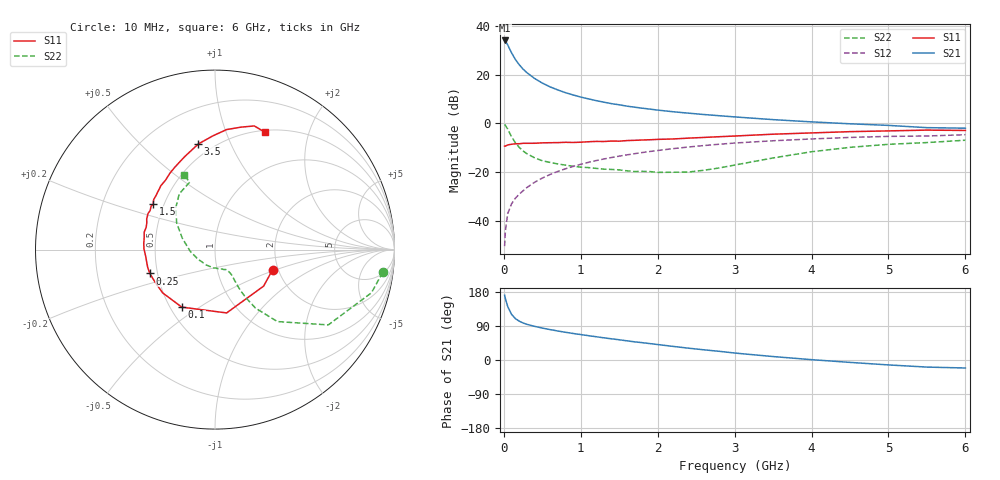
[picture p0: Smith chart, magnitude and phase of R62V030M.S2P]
! SIEMENS Small Signal Semiconductors
! BFR193
! Si NPN RF Bipolar Junction Transistor in SOT23
! VCE = 2 V  IC = 30 mA
! Common Emitter S-Parameters:  May  1996
# GHz  S  MA  R  50
!  f  S11  S21  S12  S22
! GHz  MAG  ANG  MAG  ANG  MAG  ANG  MAG  ANG
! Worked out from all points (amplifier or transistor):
!   36 points, 10 MHz to 6 GHz, reference 50 ohm
!   highest |S21| = 34.0 dB at 10 MHz (marker M1)
!   |S21| within 3 dB of that: start of sweep to 68.44 MHz
!   unconditionally stable (mu >= 1): 437.2 MHz to 1.916 GHz
!   at 250 MHz: K = 0.91, MSG = 25.0 dB, |S12| = -27.7 dB
!   at 1.4 GHz: K = 1.02, MAG = 10.1 dB, |S12| = -14.1 dB
!   at 6 GHz: K = 0.95, MSG = 1.3 dB, |S12| = -4.7 dB
!   lowest NFmin = 1.90 dB at 450 MHz
!   S11 on the Smith chart (normalised r, x): 10 MHz: 1.87, -0.48; 100 MHz: 0.57, -0.43; 250 MHz: 0.45, -0.14; 1.5 GHz: 0.44, +0.27; 3.5 GHz: 0.42, +0.76; 6 GHz: 0.52, +1.38
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0.01  0.34 -19.4  49.99 170.9  0.003 83.7  0.9431 -7.7
0.02  0.3388 -36.9  48.63 162.1  0.0061 84.1  0.9044 -15.4
0.05  0.3588 -79.6  40.64 141.2  0.0139 70.3  0.7582 -33.6
0.1  0.3701 -120.0  27.93 120.6  0.0222 65.2  0.5305 -49.1
0.15  0.3785 -140.5  20.37 109.2  0.0289 65.8  0.3968 -55.3
0.2  0.3799 -151.5  15.9 102.5  0.035 68.0  0.3194 -57.3
0.25  0.3871 -159.9  12.9 97.7  0.0411 69.3  0.2698 -58.1
0.3  0.3879 -165.4  10.9 94.1  0.048 70.4  0.2367 -58.0
0.4  0.3883 -174.9  8.291 88.8  0.0615 71.4  0.1951 -57.3
0.5  0.3958 179.4  6.673 84.3  0.0749 71.6  0.1699 -56.7
0.6  0.3984 175.1  5.586 80.3  0.0887 71.3  0.1571 -57.1
0.7  0.4003 170.1  4.832 76.6  0.1025 71.1  0.1463 -57.9
0.8  0.4063 166.2  4.249 73.2  0.116 69.9  0.1382 -58.7
0.9  0.4031 162.0  3.806 70.0  0.1302 69.0  0.1309 -60.0
1.1  0.4171 155.8  3.162 64.2  0.1575 67.0  0.1229 -65.1
1.5  0.4284 143.5  2.39 53.4  0.2112 61.6  0.1103 -79.0
2.2  0.4755 125.3  1.72 35.9  0.3011 51.3  0.0987 -119.3
3  0.5464 107.7  1.349 18.4  0.3922 38.7  0.1385 -176.0
3.5  0.5957 99.0  1.186 9.1  0.4367 30.8  0.1939 160.5
4.5  0.6718 84.5  0.974 -6.3  0.5113 16.6  0.3201 133.0
5.5  0.7229 72.4  0.812 -18.7  0.5464 2.6  0.401 110.6
6  0.711 67.1  0.791 -21.1  0.5817 -1.5  0.4481 112.3
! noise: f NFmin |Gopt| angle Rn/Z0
0.45  1.9  0.4  180  0.09
0.9  1.95  0.43  -173  0.11
1.8  2.4  0.58  -144  0.24
